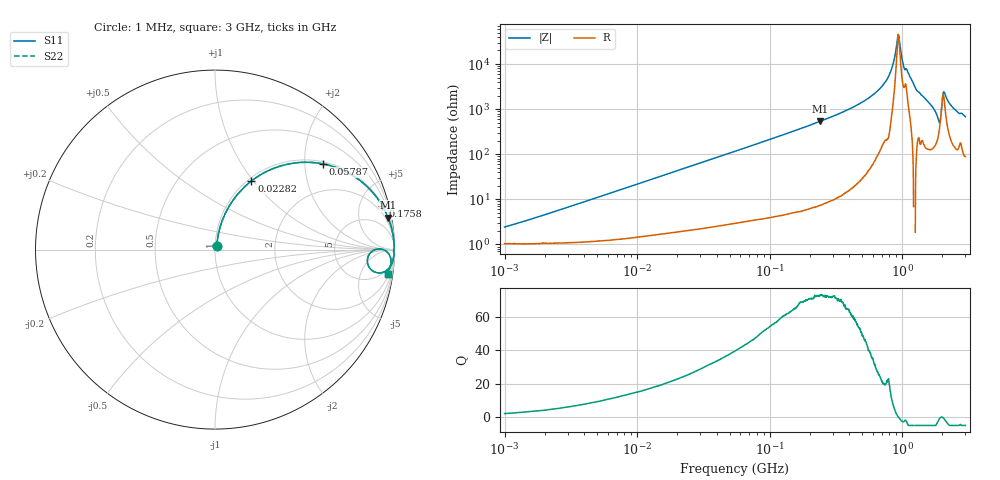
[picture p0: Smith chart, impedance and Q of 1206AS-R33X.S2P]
!s-Parameter Generated by FASTRON Sdn. Bhd.
!FASTRON P/N : 1206AS-R33X
!Keysight Technologies: E4991B_MY54100416_A.01.15
!Date created: Thu Nov 16 11:08:59 2023
!Version  : Rev00 Thu Nov 16 11:08:59 2023
!Data & Calibration Information:
!Freq	S11	S21	S12	S22
!PortZ  Port1:50+j0  Port2:50+j0
!When reading reference impedance value at option line is always used.
! Remarks : This data is being provided solely for informational purposes.
# Hz S dB R 50
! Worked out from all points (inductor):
!   1601 points, 1 MHz to 3 GHz, reference 50 ohm
!   read as one part in series: L = 352 nH near 1.405 MHz
!   highest Q = 72.8 at 240.9 MHz (marker M1), where L = 356 nH
!   self-resonance near 934.9 MHz
!   S11 on the Smith chart (normalised r, x): 1 MHz: 1.02, +0.04; 22.82 MHz: 1.04, +0.98; 57.87 MHz: 1.06, +2.46; 175.8 MHz: 1.11, +7.63; 3 GHz: 3, -13
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1000000  -32.30 63.5  -0.09 -1.3  -0.09 -1.3  -32.30 63.5
3804036  -21.59 77.6  -0.13 -4.7  -0.13 -4.7  -21.59 77.6
1.447069e7  -10.64 69.9  -0.54 -17.1  -0.54 -17.1  -10.64 69.9
2.281658e7  -7.28 62.1  -1.07 -25.6  -1.07 -25.6  -7.28 62.1
5.477226e7  -2.51 40.1  -3.83 -48.5  -3.83 -48.5  -2.51 40.1
5.787165e7  -2.31 38.6  -4.10 -50.0  -4.10 -50.0  -2.31 38.6
1.757585e8  -0.32 14.6  -11.95 -74.5  -11.95 -74.5  -0.32 14.6
2.083556e8  -0.23 12.3  -13.45 -76.9  -13.45 -76.9  -0.23 12.3
2.408952e8  -0.17 10.5  -14.79 -78.7  -14.79 -78.7  -0.17 10.5
5.418594e8  -0.03 3.4  -24.44 -85.2  -24.44 -85.2  -0.03 3.4
6.855309e8  -0.02 1.9  -29.39 -85.6  -29.39 -85.6  -0.02 1.9
7.925923e8  -0.01 1.1  -34.73 -86.3  -34.73 -86.3  -0.01 1.1
8.543737e8  -0.01 0.6  -40.01 -81.7  -40.01 -81.7  -0.01 0.6
9.117997e8  -0.02 0.2  -49.14 -54.7  -49.14 -54.7  -0.02 0.2
9.395906e8  -0.02 -0.0  -52.84 8.3  -52.84 8.3  -0.02 -0.0
1.02815e9  -0.04 -0.6  -38.89 68.9  -38.89 68.9  -0.04 -0.6
1.249715e9  -0.00 -1.9  -29.73 88.5  -29.73 88.5  -0.00 -1.9
1.86495e9  -0.60 -8.0  -16.48 59.6  -16.48 59.6  -0.60 -8.0
1.921792e9  -1.36 -5.6  -15.37 29.2  -15.37 29.2  -1.36 -5.6
2.092429e9  -0.22 -2.1  -27.27 53.8  -27.27 53.8  -0.22 -2.1
2.431346e9  -0.16 -5.2  -20.70 76.3  -20.70 76.3  -0.16 -5.2
3e9  -0.26 -8.2  -16.88 74.3  -16.88 74.3  -0.26 -8.2
